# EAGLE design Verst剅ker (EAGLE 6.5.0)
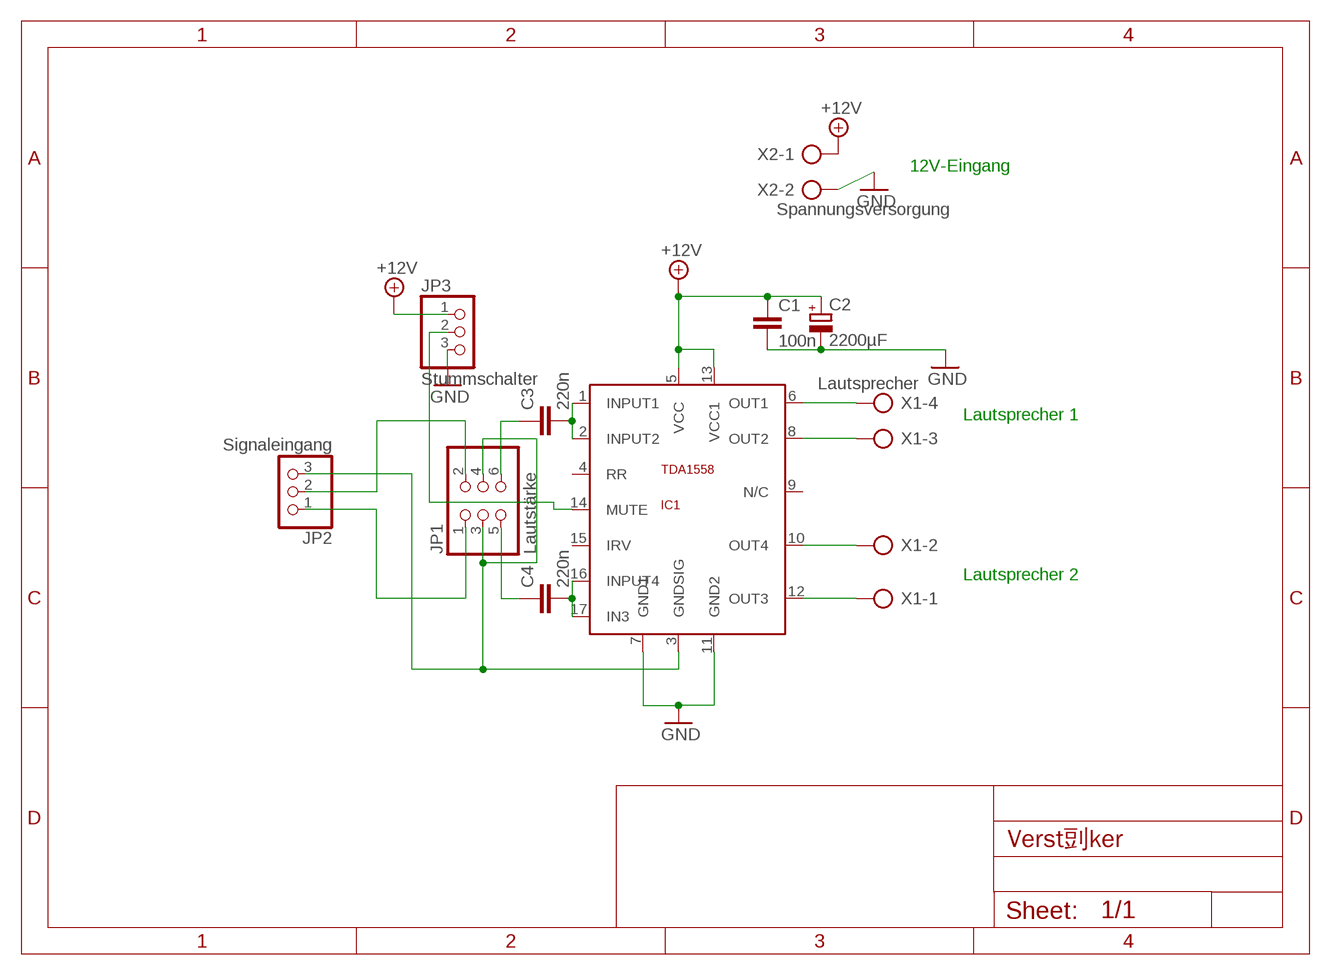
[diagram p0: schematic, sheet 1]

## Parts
C1  100n  C-EU025-024X044  [C025-024X044]
C2  2200µF  CPOL-EUE5-8.5  [E5-8,5]
C3  220n  C-EU025-024X044  [C025-024X044]
C4  220n  C-EU025-024X044  [C025-024X044]
IC1  TDA1558  TDA1558Q  [SOT243-1]
JP1  Lautstärke  PINHD-2X3  [2X03]
JP2  Signaleingang  PINHD-1X3  [1X03]
JP3  Stummschalter  PINHD-1X3  [1X03]
X1  Lautsprecher  AK300/4  [AK300/4]
X2  Spannungsversorgung  AK300/2  [AK300/2]

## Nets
+12V: C1.1 C2.+ IC1.5(VCC) IC1.13(VCC1) JP3.1 X2.1
GND: C1.2 C2.- IC1.7(GND1) IC1.11(GND2) JP3.3 X2.2
N$1: C3.2 IC1.1(INPUT1) IC1.2(INPUT2)
N$2: C4.2 IC1.16(INPUT4) IC1.17(IN3)
N$3: JP1.2 JP2.2
N$4: JP1.1 JP2.1
N$5: IC1.6(OUT1) X1.4
N$6: IC1.8(OUT2) X1.3
N$7: IC1.3(GNDSIG) JP1.3 JP1.4 JP2.3
N$8: IC1.10(OUT4) X1.2
N$9: IC1.12(OUT3) X1.1
N$10: C4.1 JP1.5
N$11: C3.1 JP1.6
N$12: IC1.14(MUTE) JP3.2
Unconnected: IC1.4(RR) IC1.9(N/C) IC1.15(IRV)

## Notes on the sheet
- 12V-Eingang
- Lautsprecher 1
- Lautsprecher 2

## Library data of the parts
C1 C3 C4 = rcl:C-EU: CAPACITOR, European symbol
C2 = rcl:CPOL-EU: POLARIZED CAPACITOR, European symbol
IC1 = Audio-Power-amplifier:TDA1558Q: http://www.datasheetcatalog.com/datasheets_pdf/T/D/A/1/TDA1558.shtml
JP1 = pinhead:PINHD-2X3: PIN HEADER
JP2 JP3 = pinhead:PINHD-1X3: PIN HEADER
X1 = con-ptr500:AK300/4: CONNECTOR; OC_FARNELL: unknown; OC_NEWARK: unknown
X2 = con-ptr500:AK300/2: CONNECTOR; OC_FARNELL: unknown; OC_NEWARK: unknown

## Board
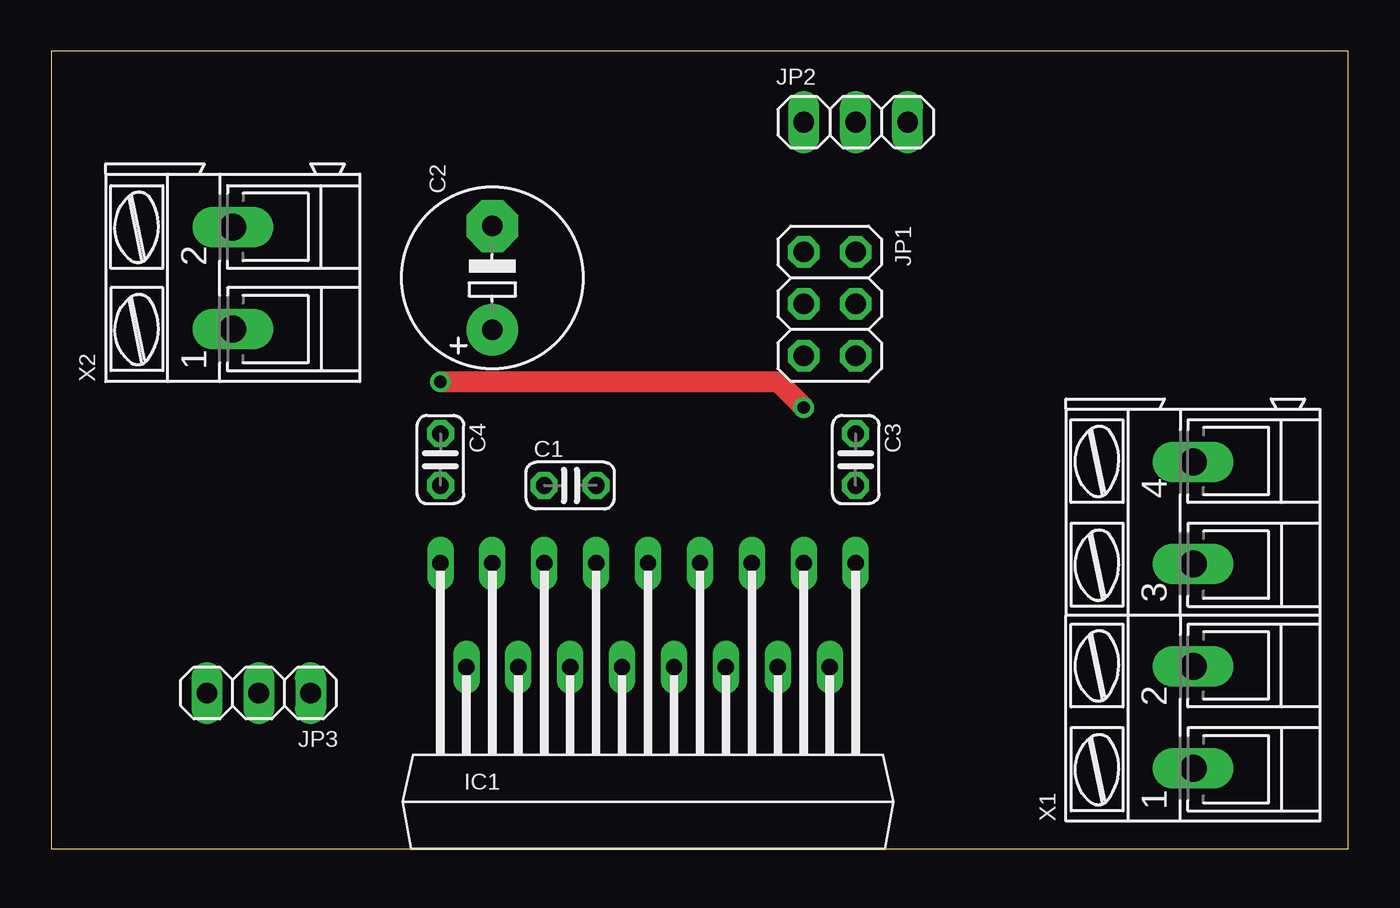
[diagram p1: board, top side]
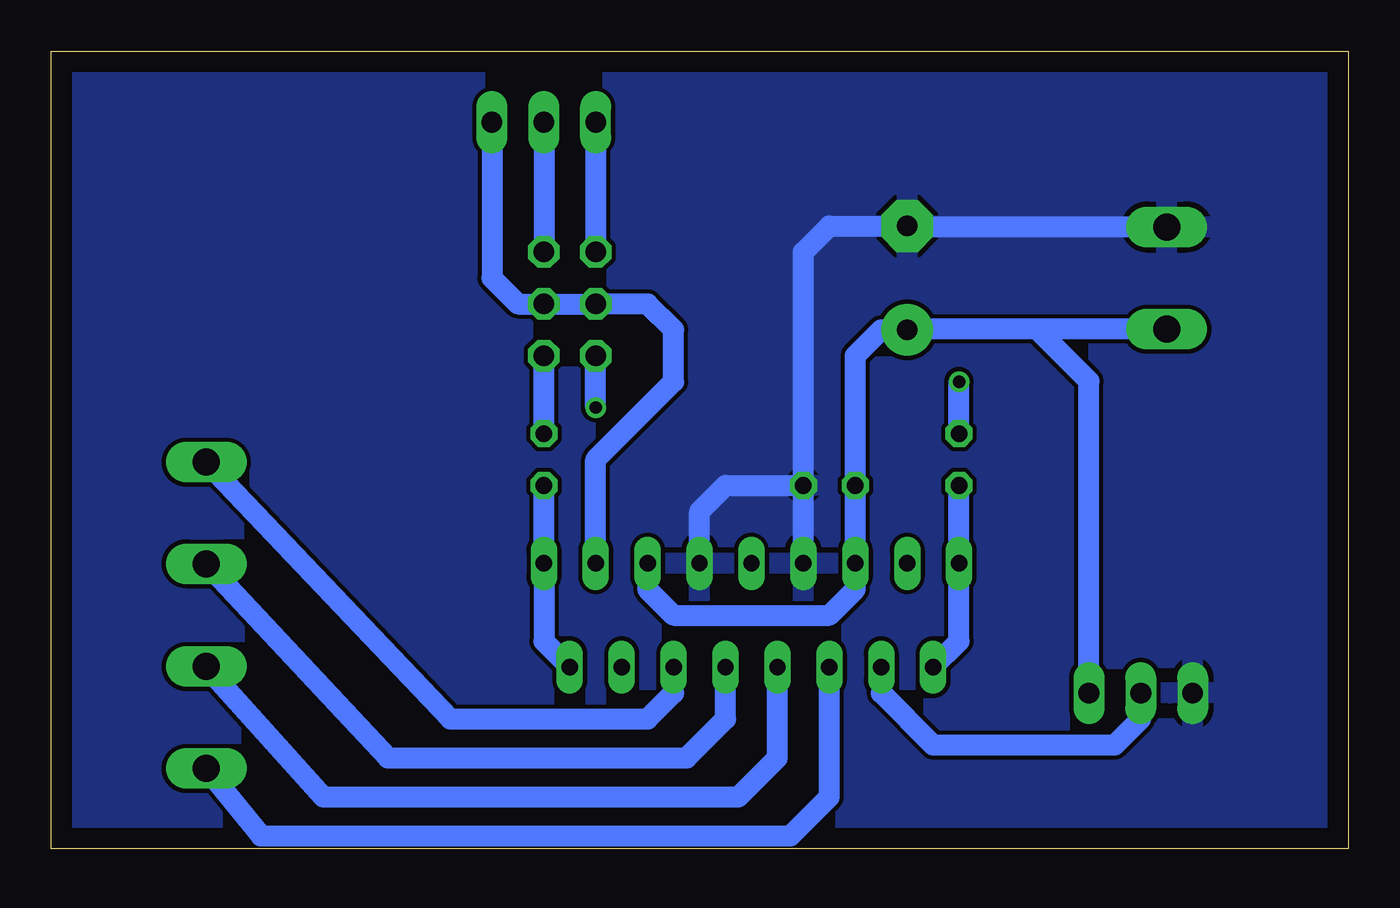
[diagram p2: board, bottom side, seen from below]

Size 63.48 x 39.04 mm. Coordinates in mm from the lower left corner, seen from the top.
Outline: 0,0 63.48,0 63.48,39.04 0,39.04 0,0
Copper layers (1*16): Top 0.035mm / dielectric 1.5mm / Bottom 0.035mm
Design rules "default": minimum track width 10mil, minimum drill 24mil, track to track 8mil, track to pad 8mil, pad to pad 8mil, via to via 8mil, smd to smd 8mil, copper to edge 40mil, drill to drill 8mil, minimum pad ring 10mil, minimum via ring 8mil, stop-mask expansion 4mil, vias tented up to drill 0mil, thermal gap 10mil

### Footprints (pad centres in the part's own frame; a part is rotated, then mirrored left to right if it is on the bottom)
C025-024X044 = drill 0.813 octagon: 1 -1.27,0; 2 1.27,0
E5-8,5 = drill 1.016 pad 2.54: + -2.54,0 | drill 1.016 pad 2.54 octagon: - 2.54,0
SOT243-1 = drill 0.8 long: 1 10.16,13.97; 2 8.89,8.89; 3 7.62,13.97; 4 6.35,8.89; 5 5.08,13.97; 6 3.81,8.89; 7 2.54,13.97; 8 1.27,8.89; 9 0,13.97; 10 -1.27,8.89; 11 -2.54,13.97; 12 -3.81,8.89; 13 -5.08,13.97; 14 -6.35,8.89; 15 -7.62,13.97; 16 -8.89,8.89; 17 -10.16,13.97
2X03 = drill 1.016 octagon: 1 -2.54,-1.27; 2 -2.54,1.27; 3 0,-1.27; 4 0,1.27; 5 2.54,-1.27; 6 2.54,1.27
1X03 = drill 1.016 long: 1 -2.54,0; 2 0,0; 3 2.54,0
AK300/4 = drill 1.321 long: 1 -7.493,0; 2 -2.515,0; 3 2.515,0; 4 7.493,0
AK300/2 = drill 1.321 long: 1 -2.515,0; 2 2.489,0

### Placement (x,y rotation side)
C1  25.4,17.78 0 top
C2  21.59,27.94 90 top
C3  39.37,19.05 270 top
C4  19.05,19.05 270 top
IC1  29.21,0 0 top
JP1  38.1,26.67 270 top
JP2  39.37,35.56 0 top
JP3  10.16,7.62 180 top
X1  55.88,11.43 90 top
X2  8.89,27.94 90 top

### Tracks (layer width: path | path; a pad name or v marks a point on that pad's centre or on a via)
+12V
  Bottom 1.016: X2.1 15.24,25.43 | 15.24,25.43 21.57,25.43 C2.+ 22.86,25.4 24.13,24.13 C1.1 IC1.13 24.13,12.7 25.4,11.43 33.02,11.43 34.29,12.7 IC1.5 | JP3.1 12.7,22.89 15.24,25.43
GND
  Bottom 1.016: X2.2 21.54,30.43 C2.- 25.4,30.48 26.67,29.21 C1.2 | IC1.11 C1.2 | IC1.7 31.75,16.51 30.48,17.78 C1.2
  pour Bottom: 0,0 63.5,0 63.5,39.37 0,39.37
N$1
  Bottom 1.016: C3.2 IC1.1 39.37,10.16 IC1.2
N$2
  Bottom 1.016: C4.2 IC1.17 19.05,10.16 IC1.16
N$3
  Bottom 1.016: JP2.2 JP1.2
N$4
  Bottom 1.016: JP2.1 JP1.1
N$5
  Bottom 1.016: X1.4 43.94,6.35 34.29,6.35 33.02,7.62 IC1.6
N$6
  Bottom 1.016: X1.3 55.85,13.97 55.88,13.97 46.99,4.45 32.38,4.45 30.48,6.35 IC1.8
N$7
  Bottom 1.016: JP2.3 41.91,27.94 40.64,26.67 JP1.4 JP1.3 34.29,26.67 33.02,25.4 33.02,22.86 36.83,19.05 IC1.3
N$8
  Bottom 1.016: X1.2 55.85,8.89 55.88,8.89 50.16,2.54 29.84,2.54 27.94,4.45 IC1.10
N$9
  Bottom 1.016: X1.1 53.21,0.64 27.3,0.64 25.4,2.54 IC1.12
N$10  (via drill 0.6)
  Top 1.016: v19.05,22.86 35.56,22.86 v36.83,21.59
  Bottom 1.016: C4.1 v19.05,22.86 | v36.83,21.59 JP1.5
N$11
  Bottom 1.016: C3.1 JP1.6
N$12
  Bottom 1.016: IC1.14 22.86,7.62 20.32,5.08 11.43,5.08 10.16,6.35 JP3.2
